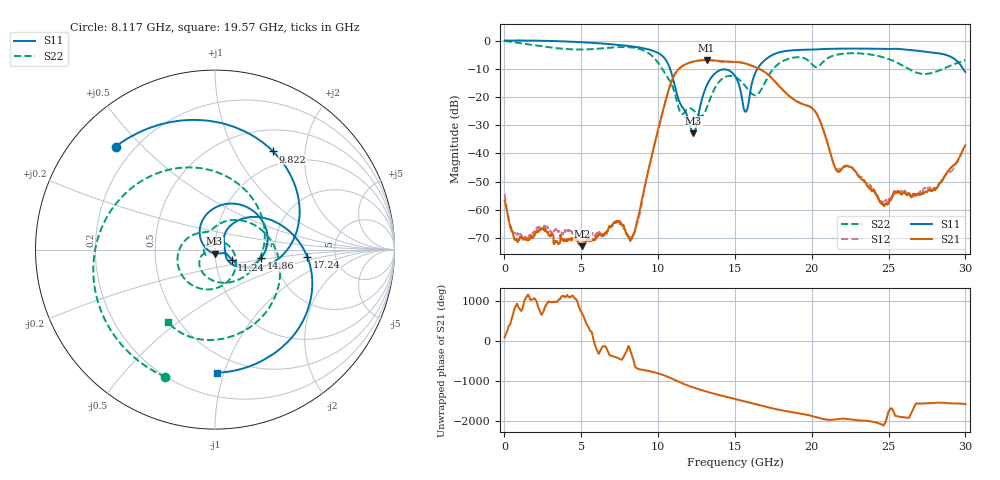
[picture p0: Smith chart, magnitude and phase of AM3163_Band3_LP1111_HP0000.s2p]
!Agilent Technologies,E8364B,MY43040894,A.07.50.67
!Agilent E8364B: A.07.50.67
!Date: Thursday, August 20, 2020 12:11:06
!Correction: S11(Full 2 Port(1,2))
!S21(Full 2 Port(1,2))
!S12(Full 2 Port(1,2))
!S22(Full 2 Port(1,2))
!S2P File: Measurements: S11, S21, S12, S22:
# Hz S  dB  R 50
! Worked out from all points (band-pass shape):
!   3201 points, 10 MHz to 30 GHz, reference 50 ohm
!   highest |S21| = -6.94 dB at 13.16 GHz (marker M1); lowest = -72.9 dB at 5.061 GHz (marker M2)
!   |S21| within 3 dB of the highest: 11.37 GHz to 16.54 GHz (5.169 GHz wide, 37 % of centre)
!   lowest |S11| = -32.9 dB at 12.29 GHz (marker M3), VSWR 1.05, Z = 49.7 - j2.25 ohm
!   |S11| at or under -10 dB: 10.78 GHz to 16.47 GHz (5.691 GHz wide, 41.8 % of centre); 29.84 GHz to end of sweep
!   |S22| runs from -26.8 to -0.2 dB; largest |S21 - S12| = 0.013
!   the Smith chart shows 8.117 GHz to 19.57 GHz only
!   S11 on the Smith chart (normalised r, x): 8.117 GHz: 0.13, +0.42; 9.822 GHz: 0.79, +1.45; 11.24 GHz: 1.20, -0.14; 14.86 GHz: 1.69, -0.16; 17.24 GHz: 3.09, -0.33; 19.57 GHz: 0.37, -0.95
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1e7  0.02 -2.1  -56.69 99.6  -54.36 19.0  -0.15 -5.0
1.247088e9  -0.01 -34.2  -70.42 -137.4  -69.70 120.7  -1.12 -82.7
2.652869e9  -0.11 -72.6  -66.75 147.5  -65.85 41.0  -2.23 -163.1
5.014581e9  -0.61 -135.6  -72.57 5.5  -70.56 -151.8  -3.20 71.5
5.061441e9  -0.62 -136.9  -72.88 -30.4  -71.03 133.2  -3.20 69.0
6.570312e9  -1.15 -178.2  -68.13 -123.3  -68.28 -96.2  -2.70 -16.4
8.116672e9  -1.96 134.0  -69.85 -152.3  -70.04 140.1  -2.37 -111.3
9.822353e9  -3.94 59.3  -35.57 -61.5  -35.62 -61.4  -6.66 101.4
1.000979e10  -4.43 47.6  -31.40 -81.5  -31.48 -81.4  -7.95 75.8
1.123751e10  -19.26 -31.1  -10.74 84.9  -10.78 85.4  -21.85 -155.9
1.228716e10  -32.87 -96.4  -7.46 -72.5  -7.46 -72.2  -24.65 175.5
1.315874e10  -16.05 120.7  -6.94 -177.5  -6.94 -178.0  -23.98 38.9
1.486442e10  -11.62 -9.9  -7.56 11.7  -7.67 13.3  -12.66 -143.1
1.5005e10  -12.57 -19.5  -7.60 -1.7  -7.65 -0.0  -12.93 -154.8
1.571726e10  -25.21 12.0  -8.22 -71.0  -8.17 -70.3  -16.41 148.4
1.723551e10  -5.75 -4.4  -12.48 142.7  -12.38 143.7  -12.05 35.6
1.95691e10  -3.26 -88.9  -22.86 -26.5  -22.73 -25.7  -6.38 -122.9
2.000958e10  -3.19 -100.2  -23.92 -67.1  -23.75 -66.8  -8.41 -137.4
2.162154e10  -2.91 -137.9  -46.14 -147.7  -45.56 -148.7  -5.05 -161.0
2.500479e10  -2.98 144.1  -57.55 44.1  -56.36 -22.5  -6.56 67.5
2.740399e10  -3.95 76.1  -53.54 -109.4  -52.34 -103.5  -11.85 -87.9
3e10  -11.15 -31.4  -37.13 -131.0  -37.81 -128.9  -6.99 130.5
